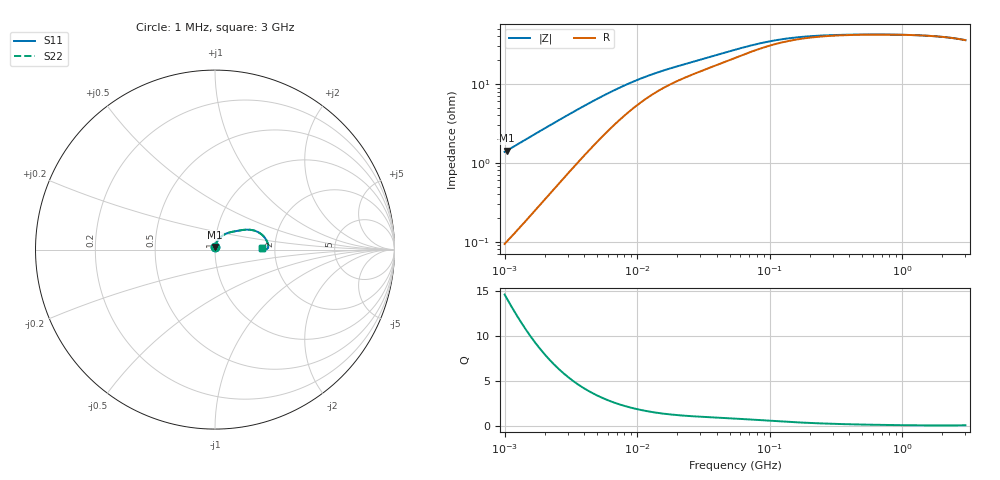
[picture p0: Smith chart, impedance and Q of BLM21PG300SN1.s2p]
! BLM21PG300SN1
# Hz S RI R 50
!Freq.(Hz) S11(Real) S11(Imag) S21(Real) S21(Imag) S12(Real) S12(Imag) S22(Real) S22(Imag)
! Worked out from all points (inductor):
!   401 points, 1 MHz to 3 GHz, reference 50 ohm
!   read as one part in series: L = 217 nH near 1.041 MHz
!   highest Q = 14.1 at 1.041 MHz (marker M1), where L = 218 nH
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1000000  0.00113 0.0137  0.9989 -0.0137  0.9989 -0.0137  0.00113 0.0137
1040844  0.00121 0.0142  0.9988 -0.0142  0.9988 -0.0142  0.00121 0.0142
2271982  0.00523 0.0303  0.9948 -0.0303  0.9948 -0.0303  0.00523 0.0303
3823119  0.0137 0.0481  0.9863 -0.0481  0.9863 -0.0481  0.0137 0.0481
5592179  0.0262 0.0644  0.9738 -0.0644  0.9738 -0.0644  0.0262 0.0644
7703107  0.0424 0.0782  0.9576 -0.0782  0.9576 -0.0782  0.0424 0.0782
9040831  0.0524 0.0843  0.9476 -0.0843  0.9476 -0.0843  0.0524 0.0843
1.061086e7  0.0633 0.0895  0.9367 -0.0895  0.9367 -0.0895  0.0633 0.0895
1.461624e7  0.0866 0.097  0.9134 -0.097  0.9134 -0.097  0.0866 0.097
2.225279e7  0.1171 0.1031  0.8829 -0.1031  0.8829 -0.1031  0.1171 0.1031
3.597591e7  0.1536 0.1092  0.8464 -0.1092  0.8464 -0.1092  0.1536 0.1092
5.477226e7  0.1912 0.1108  0.8088 -0.1108  0.8088 -0.1108  0.1912 0.1108
7.697298e7  0.2233 0.1045  0.7767 -0.1045  0.7767 -0.1045  0.2233 0.1045
1.039275e8  0.2485 0.0926  0.7515 -0.0926  0.7515 -0.0926  0.2485 0.0926
1.431579e8  0.2689 0.076  0.7311 -0.076  0.7311 -0.076  0.2689 0.076
2.094008e8  0.2841 0.0562  0.7159 -0.0562  0.7159 -0.0562  0.2841 0.0562
3.817355e8  0.2947 0.0316  0.7053 -0.0316  0.7053 -0.0316  0.2947 0.0316
8.005644e8  0.2964 0.013  0.7036 -0.013  0.7036 -0.013  0.2964 0.013
1.218836e9  0.2933 0.00653  0.7067 -0.00653  0.7067 -0.00653  0.2933 0.00653
1.712864e9  0.2873 0.00331  0.7127 -0.00331  0.7127 -0.00331  0.2873 0.00331
2.266846e9  0.2783 0.00304  0.7217 -0.00304  0.7217 -0.00304  0.2783 0.00304
3e9  0.2638 0.00727  0.7362 -0.00727  0.7362 -0.00727  0.2638 0.00727
